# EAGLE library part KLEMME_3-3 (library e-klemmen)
Klemme 3 3
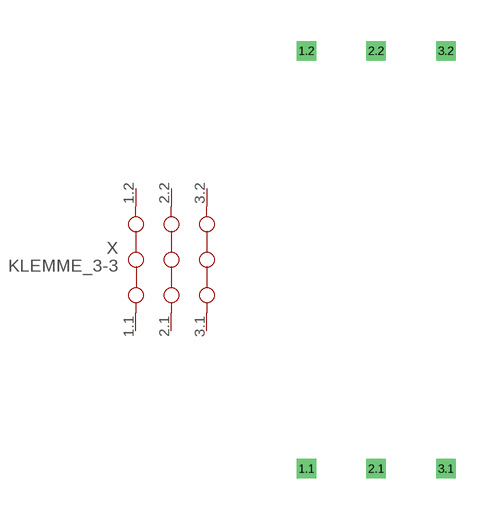
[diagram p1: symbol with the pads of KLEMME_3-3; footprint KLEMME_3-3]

Designator prefix X

## KLEMME_3-3  [KLEMME_3-3]
1.1  1.1  pas
1.2  1.2  pas
2.1  2.1  pas
2.2  2.2  pas
3.1  3.1  pas
3.2  3.2  pas

## Footprint KLEMME_3-3 (pad centres in mm)
Dummy
drill 0.2 pad 0.6 square: 1.1 -2.54,-7.62; 1.2 -2.54,7.62; 2.1 0,-7.62; 2.2 0,7.62; 3.1 2.54,-7.62; 3.2 2.54,7.62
